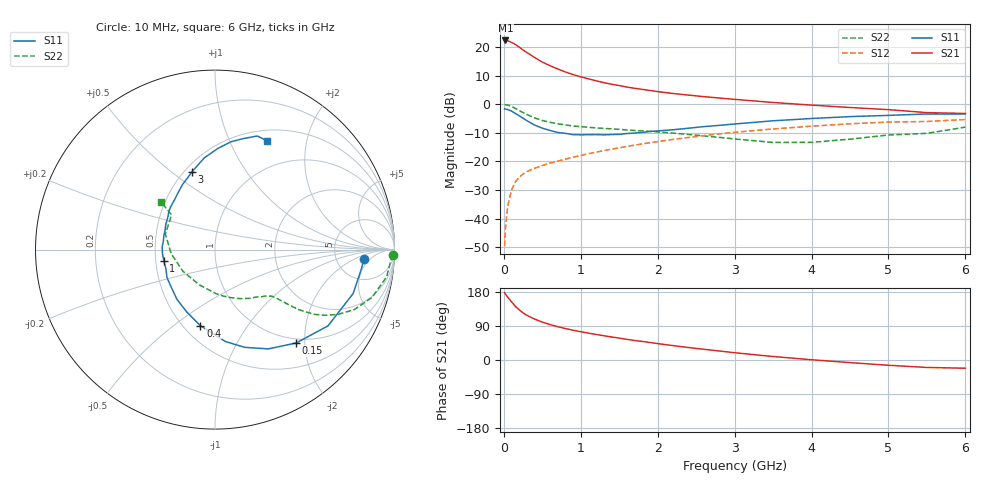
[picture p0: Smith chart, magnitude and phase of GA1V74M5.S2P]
! Infineon Technologies  Discrete & RF Semiconductors
! BF775
! Si NPN RF Bipolar Junction Transistor in SOT23
! VCE = 1.75 V  IC = 4.5 mA
! Common Emitter S-Parameters:  May  1996
# GHz  S  MA  R  50
!  f  S11  S21  S12  S22
! GHz  MAG  ANG  MAG  ANG  MAG  ANG  MAG  ANG
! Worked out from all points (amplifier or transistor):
!   36 points, 10 MHz to 6 GHz, reference 50 ohm
!   highest |S21| = 22.3 dB at 20 MHz (marker M1)
!   |S21| within 3 dB of that: start of sweep to 233.5 MHz
!   unconditionally stable (mu >= 1): 792 MHz to 4.175 GHz; 5.191 GHz to end of sweep
!   at 250 MHz: K = 0.47, MSG = 21.7 dB, |S12| = -24.4 dB
!   at 1.4 GHz: K = 1.15, MAG = 9.0 dB, |S12| = -15.7 dB
!   at 6 GHz: K = 1.00, MAG = 0.7 dB, |S12| = -5.3 dB
!   S11 on the Smith chart (normalised r, x): 10 MHz: 10, -3; 150 MHz: 0.92, -1.82; 400 MHz: 0.60, -0.63; 1 GHz: 0.55, -0.08; 3 GHz: 0.54, +0.59; 6 GHz: 0.63, +1.39
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0.01  0.8314 -3.5  12.98 177.4  0.0033 91.3  0.9899 -1.7
0.02  0.8234 -7.2  13.03 174.1  0.0066 85.7  0.9812 -3.6
0.05  0.8078 -17.6  12.92 166.0  0.0165 79.9  0.9683 -9.0
0.1  0.7597 -34.0  12.07 153.5  0.0316 72.1  0.9148 -16.9
0.15  0.6894 -49.0  11.08 141.3  0.0439 65.4  0.8451 -23.3
0.2  0.6278 -61.8  9.969 132.3  0.0529 61.0  0.7742 -27.8
0.25  0.5691 -73.1  8.881 124.4  0.0602 57.7  0.7129 -30.9
0.3  0.5155 -83.5  8.007 117.8  0.0665 55.3  0.6607 -33.1
0.4  0.4315 -100.9  6.572 108.0  0.076 53.1  0.5761 -35.6
0.5  0.3813 -114.4  5.455 100.0  0.0845 52.3  0.5194 -36.7
0.6  0.3484 -127.6  4.714 93.5  0.0936 52.2  0.4839 -37.3
0.8  0.3095 -149.8  3.666 83.0  0.1097 52.8  0.4344 -38.3
1  0.2919 -167.3  3.013 74.6  0.1271 53.7  0.4053 -39.7
1.1  0.2932 -175.5  2.777 71.0  0.1362 53.7  0.3952 -41.0
1.3  0.2915 171.1  2.386 64.0  0.1546 53.5  0.3782 -43.3
1.6  0.3078 153.1  1.997 54.5  0.1825 52.7  0.3547 -48.1
2.2  0.358 129.0  1.541 38.0  0.2428 49.0  0.3127 -60.9
3  0.4516 106.6  1.217 19.2  0.3232 40.7  0.2473 -87.9
3.5  0.5136 96.8  1.073 9.2  0.3698 34.5  0.2149 -114.0
4.5  0.6074 81.6  0.877 -6.9  0.455 21.4  0.245 -174.5
5.5  0.6754 69.6  0.713 -19.7  0.4989 6.8  0.3097 141.3
6  0.6721 64.5  0.69 -21.7  0.5408 2.9  0.3979 138.6
